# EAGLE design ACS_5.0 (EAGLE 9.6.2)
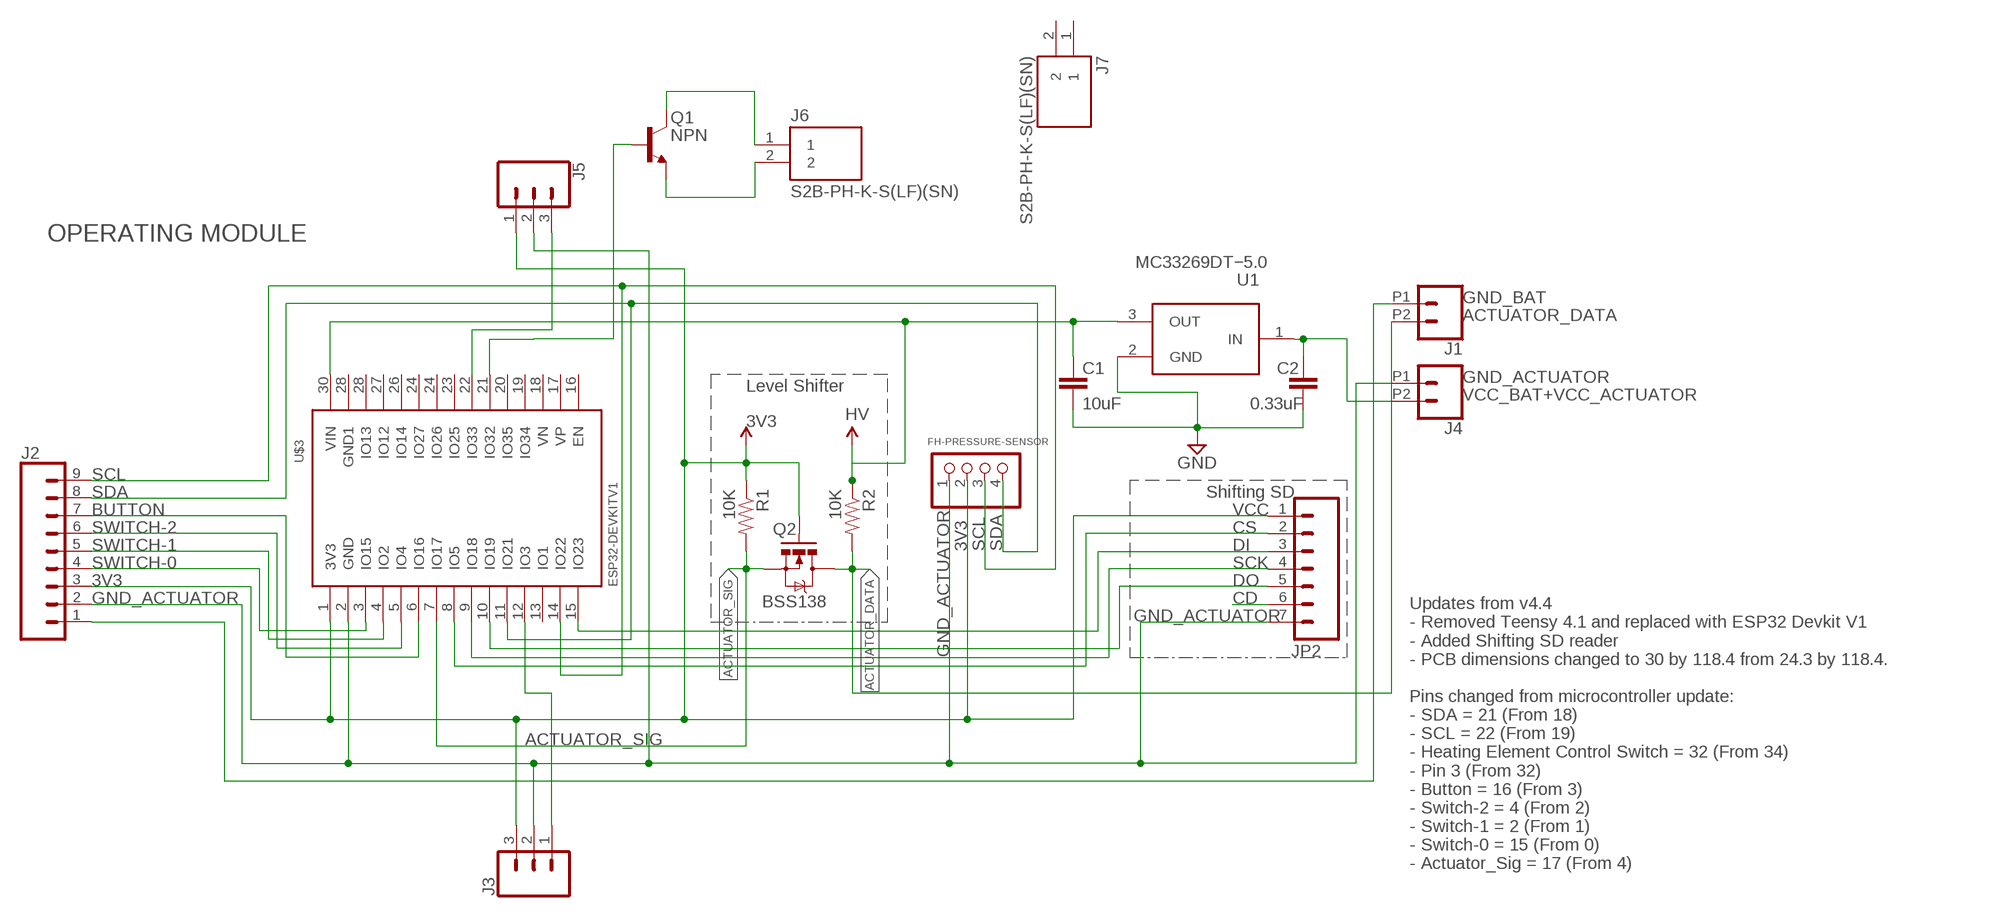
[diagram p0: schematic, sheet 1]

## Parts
C1  10uF  C_CHIP-0603(1608-METRIC)  [CAPC1608X85]
C2  0.33uF  C_CHIP-0603(1608-METRIC)  [CAPC1608X85]
FH-PRESSURE-SENSOR  PINHD-1X4  [1X04]
J1  CONN_022.54MM_SCREWTERM  [1X02_2.54_SCREWTERM]
J2  CONN_09  [1X09]
J3  CONN_03  [1X03]
J4  CONN_022.54MM_SCREWTERM  [1X02_2.54_SCREWTERM]
J5  CONN_03  [1X03]
J6  S2B-PH-K-S(LF)(SN)  [JST_S2B-PH-K-S(LF)(SN)]
J7  S2B-PH-K-S(LF)(SN)  [JST_S2B-PH-K-S(LF)(SN)]
JP2  M07  [1X07]
Q1  NPN  NPN_SOT23  [SOT95P237X112-3N]
Q2  BSS138  MOSFET-NCHANNELSMD  [SOT23-3]
R1  10K  RESISTOR0603-RES  [0603-RES]
R2  10K  RESISTOR0603-RES  [0603-RES]
U1  MC78M05BDTRKG  [MC78M05BDTRKG]
U$3  ESP32DEVKITV1  [ESP32-DEVKITV1]

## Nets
3V3: FH-PRESSURE-SENSOR.2 J2.3 J3.3 J5.1 JP2.1 Q2.1(G) R1.1 U$3.1(3V3) ; supply symbol labelled LV
ACTUATOR_DATA: J1.P2 Q2.3(D) R2.2
ACTUATOR_SIG: Q2.2(S) R1.2 U$3.7(IO17)
BUTTON: J2.7 U$3.6(IO16)
GND: C1.2 C2.2 U1.2(GND)
GND_ACTUATOR: FH-PRESSURE-SENSOR.1 J2.2 J3.2 J4.P1 J5.2 JP2.7 U$3.2(GND)
GND_BAT: J1.P1 J2.1
HV: C1.1 R2.1 U1.3(OUT) U$3.30(VIN)
N$1: J5.3 U$3.22(IO33)
N$3: J6.1 Q1.3(C)
N$4: J6.2 Q1.1(E)
N$5: Q1.2(B) U$3.21(IO32)
N$8: JP2.6
N$10: J3.1 U$3.12(IO3)
N$11: JP2.3 U$3.15(IO23)
N$12: JP2.2 U$3.8(IO5)
N$13: JP2.4 U$3.9(IO18)
N$14: JP2.5 U$3.10(IO19)
SCL: FH-PRESSURE-SENSOR.3 J2.9 U$3.14(IO22)
SDA: FH-PRESSURE-SENSOR.4 J2.8 U$3.11(IO21)
SWITCH-0: J2.4 U$3.3(IO15)
SWITCH-1: J2.5 U$3.4(IO2)
SWITCH-2: J2.6 U$3.5(IO4)
VCC_BAT+VCC_ACTUATOR: C2.1 J4.P2 U1.1(IN)
Unconnected: J7.1 J7.2 U$3.13(IO1) U$3.16(EN) U$3.17(VP) U$3.18(VN) U$3.19(IO34) U$3.20(IO35) U$3.23(IO25) U$3.24(IO26) U$3.24(IO27) U$3.26(IO14) U$3.27(IO12) U$3.28(GND1) U$3.28(IO13)

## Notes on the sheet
- Heating Element 
  Control Switch
- OPERATING MODULE
- Actuator Voltage: 7.5 MAX
- MC33269DT−5.0
- Level Shifter
- Shifting SD
- VCC
- CS
- DI
- SCK
- DO
- CD
- Updates from v4.4
  - Removed Teensy 4.1 and replaced with ESP32 Devkit V1
  - Added Shifting SD reader
  - PCB dimensions changed to 30 by 118.4 from 24.3 by 118.4.
  
  Pins changed from microcontroller update:
  - SDA = 21 (From 18)
  - SCL = 22 (From 19)
  - Heating Element Control Switch = 32 (From 34)
  - Pin 3 (From 32)
  - Button = 16 (From 3)
  - Switch-2 = 4 (From 2)
  - Switch-1 = 2 (From 1)
  - Switch-0 = 15 (From 0)
  - Actuator_Sig = 17 (From 4)

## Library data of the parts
C1 C2 = Capacitor:C: Capacitor - Generic; CATEGORY: Capacitor
FH-PRESSURE-SENSOR = pinhead:PINHD-1X4: PIN HEADER
J1 J4 = SparkFun-Connectors:CONN_02: Multi connection point. Often used as Generic Header-pin footprint for 0.1 inch spaced/style header connections
J2 = SparkFun-Connectors:CONN_09: Multi connection point. Often used as Generic Header-pin footprint for 0.1 inch spaced/style header connections On any of the 0.1 inch spaced packages, you can populate with these: Break Away Headers - Straight (PRT-00116) Break Away Male Headers - Right Angle (PRT-00553) Female Headers (PRT-00115)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
J3 J5 = SparkFun-Connectors:CONN_03: Multi connection point. Often used as Generic Header-pin footprint for 0.1 inch spaced/style header connections On any of the 0.1 inch spaced packages, you can populate with these: Break Away Headers - Straight (PRT-00116) Break Away Male Headers - Right Angle (PRT-00553) Female Headers (PRT-00115)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
J6 J7 = S2B-PH-K-S_LF__SN_:S2B-PH-K-S(LF)(SN): PH Series 2 Position 2.0 mm Through Hole Side Entry Shrouded Header Check availability; AVAILABILITY: In Stock; DESCRIPTION: Connector Header Through Hole, Right Angle 2 position; MF: JST Sales America Inc.; MP: S2B-PH-K-S(LF)(SN); PACKAGE: None; PRICE: None; PURCHASE-URL: https://pricing.snapeda.com/search/part/S2B-PH-K-S(LF)(SN)/?ref=eda
JP2 = SparkFun-Connectors:M07: Header 7 Standard 7-pin 0.1" header. Use with straight break away headers (SKU : PRT-00116), right angle break away headers (PRT-00553), swiss pins (PRT-00743), machine pins (PRT-00117), and female headers (PRT-00115). NOTES ON THE VARIANTS LOCK and LOCK_LONGPADS... This footprint was designed to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
Q1 = Transistor:NPN: NPN - Generic; CATEGORY: Transistor; SUB-CATEGORY: BJT; TYPE: NPN
Q2 = SparkFun:MOSFET-NCHANNEL
R1 R2 = SparkFun:RESISTOR: Resistor
U1 = LDO:MC78M05BDTRKG: IC REG LINEAR 5V 500MA DPAK Manufacturer's datasheet; CREATED_BY: PCBLayout.com; DIGIKEY_PN: MC78M05BDTRKGOSCT-ND; MANUFACTURER: ON Semiconductor; MPN: IC REG LINEAR 5V 500MA DPAK; PACKAGE: DPak
U$3 = ESP32-DEVKITV1:ESP32DEVKITV1

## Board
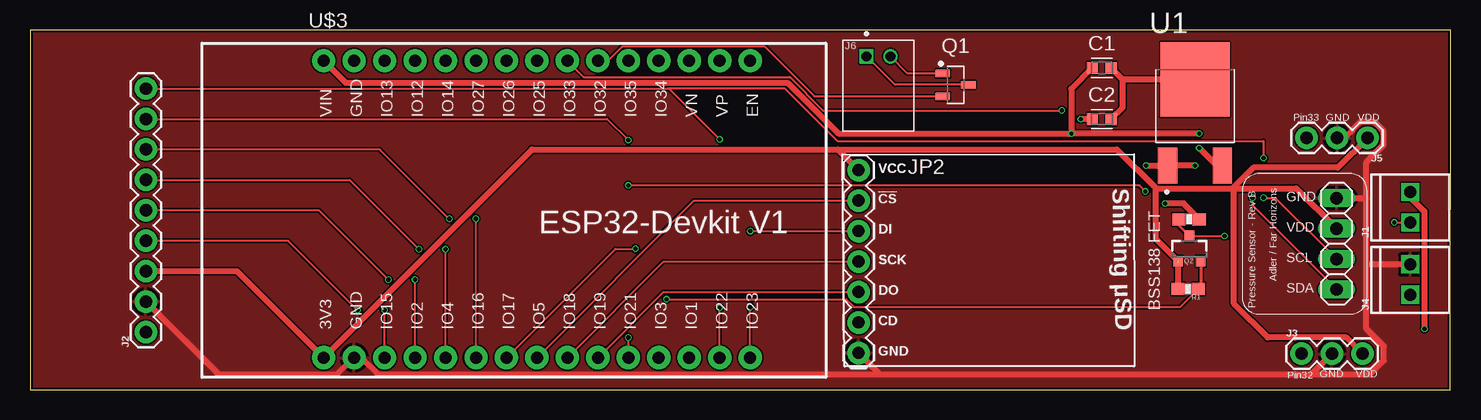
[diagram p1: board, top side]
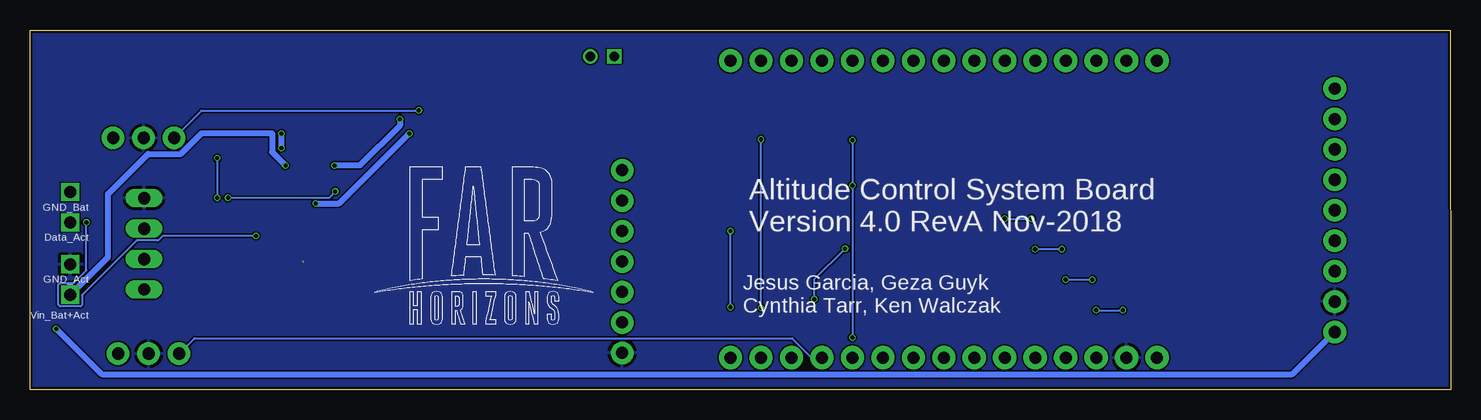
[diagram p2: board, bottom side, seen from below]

Size 118.43 x 30 mm. Coordinates in mm from the lower left corner, seen from the top.
Outline: 0,0 118.4,0 118.43,30 0.03,30 0,0
Copper layers (1*16): Top 0.035559375mm / dielectric 1.6mm / Bottom 0.035559375mm
Design rules "jlcpcb2layer": minimum track width 5mil, minimum drill 12mil, track to track 5mil, track to pad 5mil, pad to pad 5mil, via to via 5mil, smd to smd 5mil, copper to edge 8mil, drill to drill 6mil, minimum pad ring 5mil, minimum via ring 3mil, stop-mask expansion 2.5mil, vias tented up to drill 0mil, thermal gap 10mil

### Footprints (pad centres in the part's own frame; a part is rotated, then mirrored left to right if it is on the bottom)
CAPC1608X85 = smd 0.921 x 0.97: 1 -0.775,0; 2 0.775,0
1X04 = drill 1.016 long: 1 -3.81,0; 2 -1.27,0; 3 1.27,0; 4 3.81,0
1X02_2.54_SCREWTERM = drill 1.016 square: P1 2.54,0; P2 0,0
1X09 = drill 1.016 pad 1.88: 1 0,0; 2 2.54,0; 3 5.08,0; 4 7.62,0; 5 10.16,0; 6 12.7,0; 7 15.24,0; 8 17.78,0; 9 20.32,0
1X03 = drill 1.016 pad 1.88: 1 0,0; 2 2.54,0; 3 5.08,0
JST_S2B-PH-K-S(LF)(SN) = drill 0.8 square: 1 -1,0 | drill 0.8: 2 1,0
1X07 = drill 1.016 pad 1.88: 1 0,0; 2 2.54,0; 3 5.08,0; 4 7.62,0; 5 10.16,0; 6 12.7,0; 7 15.24,0
SOT95P237X112-3N = smd 1.224 x 0.625: 1 -1.064,0.95; 2 -1.064,-0.95; 3 1.064,0
SOT23-3 = smd 0.8 x 0.9: 1 -0.95,-1; 2 0.95,-1; 3 0,1.1
0603-RES = smd 1.1 x 1: 1 -0.85,0; 2 0.85,0
MC78M05BDTRKG = smd 1.6 x 3: 1 -2.285,-4.08; 3 2.285,-4.08 | smd 5.8 x 6.2: 2 0,3.1
ESP32-DEVKITV1 = drill 1 pad 1.93: 1 -22.87,-13.54; 2 -20.33,-13.54; 3 -17.79,-13.54; 4 -15.25,-13.54; 5 -12.71,-13.54; 6 -10.17,-13.54; 7 -7.63,-13.54; 8 -5.09,-13.54; 9 -2.55,-13.54; 10 -0.01,-13.54; 11 2.53,-13.54; 12 5.07,-13.54; 13 7.61,-13.54; 14 10.15,-13.54; 15 12.69,-13.54; 16 12.69,11.23; 17 10.15,11.23; 18 7.61,11.23; 19 5.07,11.23; 20 2.53,11.23; 21 -0.01,11.23; 22 -2.55,11.23; 23 -5.09,11.23; 24 -7.63,11.23; 25 -10.17,11.23; 26 -12.71,11.23; 27 -15.25,11.23; 28 -17.79,11.23; 29 -20.33,11.23; 30 -22.87,11.23

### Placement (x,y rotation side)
C1  89.35,26.84 0 top
C2  89.35,22.56 0 top
FH-PRESSURE-SENSOR  108.92,12.15 270 top
J1  115.07,13.94 90 top
J2  9.66,4.79 90 top
J3  106,3 0 top
J4  115.07,7.91 90 top
J5  111.5,21 180 top
J6  70.73,27.8 0 top
J7  not placed on the board
JP2  69.07,18.3 270 top
Q1  77.16,25.42 0 top
Q2  96.65,11.72 0 top
R1  96.56,8.41 0 top
R2  96.62,14.21 180 top
U1  97.11,22.77 0 top
U$3  47.34,16.2 0 top

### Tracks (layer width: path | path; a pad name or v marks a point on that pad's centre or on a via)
3V3  (1 unrouted)
  Top 0.152: 95.7,8.42 R1.1
  Top 0.254: 95.68,10.73 Q2.1 | 95.71,10.58 95.68,10.61
  Top 0.508: J2.3 17.27,9.88 U$3.1 41.84,20.03 67.34,20.03 | JP2.1 67.34,20.03 | 67.34,20.03 90.6,20.03 93.84,16.79 93.84,16.78 | 93.84,16.78 100.37,16.78 | 93.84,16.78 93.84,12.57 Q2.1 95.7,8.41 R1.1 | 105.44,4.35 105.43,4.33 | J3.3 109.73,4.35 105.44,4.35 | J5.1 109.02,18.52 101.98,18.52 100.37,16.91 100.37,16.78 | 100.37,16.78 105.56,16.78 FH-PRESSURE-SENSOR.2 | 105.44,4.35 103.18,4.35 100.37,7.16 100.37,16.78
ACTUATOR_DATA  (via drill 0.35)
  Top 0.152: Q2.3 v99.59,12.82 | v113.73,13.95 v113.74,13.94 J1.P2
  Top 0.254: R2.2 95.77,13.7 Q2.3
  Bottom 0.152: v99.59,12.82 107.36,12.82 107.75,12.43 109.53,12.43 114.08,7.89 114.08,7.05 114.21,6.92 115.93,6.92 116.06,7.05 116.06,8.76 115.93,8.9 114.77,8.9 113.73,9.94 v113.73,13.95
ACTUATOR_SIG  (via drill 0.35)
  Top 0.152: 97.47,8.48 R1.2 95.88,6.88 68.68,6.88 68.02,7.53 v53.06,7.53 | U$3.7 48.8,11.75 v50.48,11.75
  Top 0.254: Q2.2 97.6,8.6 97.47,8.48
  Bottom 0.152: v50.48,11.75 53.06,9.17 v53.06,7.53
BUTTON  (via drill 0.35)
  Top 0.152: U$3.6 v37.17,14.25 | v34.95,14.25 29.16,20.04 J2.7
  Bottom 0.152: v37.17,14.25 v34.95,14.25
GND
  Top 0.508: U1.2 91.09,25.87 | 91.09,25.87 C1.2 | C2.2 91.09,23.53 91.09,25.87
GND_ACTUATOR
  Top 0.508: J2.2 15.73,1.27 25.62,1.27 U$3.2 27.61,2.67 29.01,1.27 70.86,1.27 | 70.86,1.27 106.81,1.27 | JP2.7 70.86,1.27 | 106.81,1.27 J3.2 | 106.81,1.27 111.7,1.27 112.86,2.43 112.86,3.6 111.4,5.06 111.4,10.61 | J4.P1 111.56,10.45 111.4,10.61 | 111.4,10.61 111.4,15.95 | 111.4,15.95 111.4,19 112.85,20.44 112.85,21.56 112.06,22.35 110.94,22.35 109.6,21 J5.2 | FH-PRESSURE-SENSOR.1 111.39,15.96 111.4,15.95
  pour Top: -4.15,31.64 -4.15,-1.81 119.4,-1.81 119.4,31.64
  pour Bottom: -5.76,31.6 -5.76,-1.75 119.61,-1.75 119.61,31.6
GND_BAT  (via drill 0.35)
  Top 0.508: J1.P1 115.07,16.04 116.25,14.86 v116.25,5.07 v116.25,5.06
  Bottom 0.508: v116.25,5.06 112.46,1.27 13.18,1.27 J2.1
HV  (via drill 0.35)
  Top 0.508: 24.48,27.43 26.31,25.6 63.13,25.6 67.38,21.36 v86.81,21.36 | 24.48,27.43 | U$3.30 24.48,27.43 | U1.3 98.92,18.69 v97.47,20.14 | v97.47,21.36 v86.81,21.36 | v86.81,21.36 86.81,25.07 C1.1 | R2.1 96.15,15.52 v94.62,15.52
  Bottom 0.508: v97.47,20.14 v97.47,21.36 | v94.62,15.52 92.64,15.52 v86.81,21.36
N$1  (via drill 0.35)
  Top 0.152: U$3.22 46.15,26.08 63.34,26.08 66.12,23.29 v86.03,23.29
  Bottom 0.152: v86.03,23.29 104.13,23.29 J5.3
N$3
  Top 0.152: Q1.3 72.11,25.42 J6.1
N$4
  Top 0.152: Q1.1 73.16,26.37 J6.2
N$5
  Top 0.152: U$3.21 48.19,27.43 49.38,28.63 61.22,28.63 65.38,24.47 Q1.2
N$10
  Bottom 0.152: U$3.12 53.27,2.67 54.89,4.29 104.71,4.29 J3.1
N$11  (via drill 0.35)
  Top 0.152: U$3.15 v60.03,6.88 | v60.03,13.22 JP2.3
  Bottom 0.152: v60.03,6.88 v60.03,13.22
N$12
  Top 0.152: U$3.8 55.35,15.76 JP2.2
N$13
  Top 0.152: U$3.9 52.81,10.68 JP2.4
N$14
  Top 0.152: U$3.10 52.81,8.14 JP2.5
SCL  (via drill 0.35)
  Top 0.152: U$3.14 v57.49,6.8 v57.49,6.81 | J2.9 53.17,25.11 53.25,25.11 | 53.25,25.11 v57.49,20.88 | v102.83,19.3 102.83,20.75 67.3,20.75 62.94,25.11 53.25,25.11 | v102.83,16 103.8,16 FH-PRESSURE-SENSOR.3
  Bottom 0.152: v57.49,6.81 v57.49,20.88 | v102.83,19.3 v102.83,16
SDA  (via drill 0.35)
  Top 0.152: J2.8 48.12,22.57 | U$3.11 v49.88,4.34 | v92.98,16.53 92.48,17.03 v49.88,17.03 | FH-PRESSURE-SENSOR.4 101.92,15.34 v101.92,16 | v49.88,20.82 48.12,22.57 | 48.12,22.57
  Bottom 0.152: v92.98,16.53 93.51,16 v101.92,16 | v49.88,20.82 v49.88,17.03 v49.88,4.34
SWITCH-0  (via drill 0.35)
  Top 0.152: U$3.3 v29.55,6.62 | v27.32,6.62 21.52,12.41 J2.4
  Bottom 0.152: v29.55,6.62 v27.32,6.62
SWITCH-1  (via drill 0.35)
  Top 0.152: U$3.4 v32.09,9.17 | v29.87,9.17 24.09,14.96 J2.5
  Bottom 0.152: v32.09,9.17 v29.87,9.17
SWITCH-2  (via drill 0.35)
  Top 0.152: U$3.5 v34.63,11.71 | J2.6 26.62,17.5 v32.41,11.71
  Bottom 0.152: v34.63,11.71 v32.41,11.71
VCC_BAT+VCC_ACTUATOR  (via drill 0.35)
  Top 0.508: v97.13,18.69 U1.1 | C2.1 v87.59,22.56 | v93.05,18.69 U1.1 | U1.1
  Bottom 0.508: J4.P2 111.91,11.07 111.91,16.33 108.59,19.65 105.86,19.65 104.13,21.39 98.25,21.39 98.25,19.82 v97.13,18.69 | v87.59,22.56 87.59,22.04 90.94,18.69 v93.05,18.69

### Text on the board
tPlace: VCC | VCC | !CS | DI | DI | SCK | SCK | Shifting µSD | DO | DO | BSS138 FET | CD | CD | GND | GND
bPlace: Altitude Control System Board / Version 4.0 RevA Nov-2018 | Jesus Garcia, Geza Guyk / Cynthia Tarr, Ken Walczak
tNames: Pin33 | GND | VDD | Pressure Sensor - Rev B | Adler / Far Horizons | GND | VDD | SCL | SDA | Pin32 | GND | VDD
bNames: GND_Bat | Data_Act | GND_Act | Vin_Bat+Act

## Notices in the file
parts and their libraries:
SparkFun-Connectors: Licensing: Creative Commons ShareAlike 4.0 International - https://creativecommons.org/licenses/by-sa/4.0
SparkFun-Connectors: Licensing: CC v3.0 Share-Alike You are welcome to use this library for commercial purposes.
